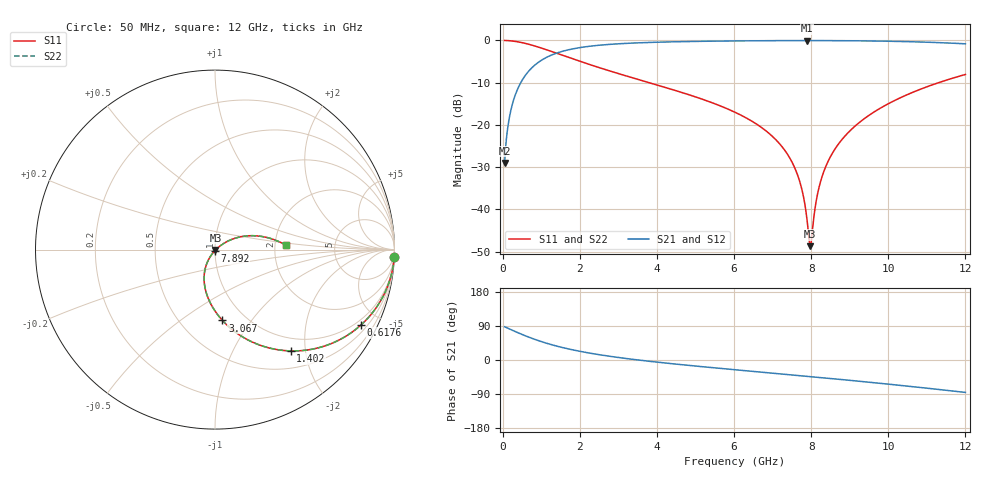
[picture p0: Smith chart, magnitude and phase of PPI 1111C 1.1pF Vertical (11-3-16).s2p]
# GHz S MA R 50
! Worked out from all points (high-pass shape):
!   1601 points, 50 MHz to 12 GHz, reference 50 ohm
!   highest |S21| = -0.04 dB at 7.892 GHz (marker M1); lowest = -29.0 dB at 50 MHz (marker M2)
!   |S21| within 3 dB of the highest: 1.389 GHz to end of sweep
!   lowest |S11| = -48.7 dB at 7.974 GHz (marker M3), VSWR 1.01, Z = 50.2 - j0.276 ohm
!   |S11| at or under -10 dB: 3.796 GHz to 11.31 GHz (7.509 GHz wide, 99.5 % of centre)
!   |S22| runs from -48.7 to 0.0 dB; largest |S21 - S12| = 0
!   S11 on the Smith chart (normalised r, x): 50 MHz: 1, -49; 617.6 MHz: 0.77, -3.98; 1.402 GHz: 0.77, -1.73; 3.067 GHz: 0.78, -0.73; 7.892 GHz: 1.00, -0.01; 12 GHz: 2.30, +0.13
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0.05  0.9994 -2.3  0.03551 87.7  0.03551 87.7  0.9994 -2.3
0.1545625  0.994 -7.2  0.1092 82.8  0.1092 82.8  0.994 -7.2
0.259125  0.9834 -11.9  0.1811 78.0  0.1811 78.0  0.9834 -11.9
0.617625  0.9152 -27.3  0.4024 62.7  0.4024 62.7  0.9152 -27.3
1.401844  0.7046 -53.2  0.7085 36.7  0.7085 36.7  0.7046 -53.2
2.044156  0.5581 -67.8  0.8283 22.1  0.8283 22.1  0.5581 -67.8
3.067375  0.3966 -84.0  0.9161 5.7  0.9161 5.7  0.3966 -84.0
4.038312  0.2934 -95.6  0.9536 -6.0  0.9536 -6.0  0.2934 -95.6
6.025  0.1411 -114.6  0.9869 -25.7  0.9869 -25.7  0.1411 -114.6
6.824156  0.08528 -121.0  0.9929 -33.1  0.9929 -33.1  0.08528 -121.0
7.361906  0.04665 -123.9  0.9952 -38.1  0.9952 -38.1  0.04665 -123.9
7.698  0.02179 -121.9  0.9958 -41.2  0.9958 -41.2  0.02179 -121.9
7.810031  0.01346 -116.8  0.9959 -42.2  0.9959 -42.2  0.01346 -116.8
7.892188  0.007586 -104.6  0.9959 -43.0  0.9959 -43.0  0.007586 -104.6
7.974344  0.003665 -48.6  0.9959 -43.8  0.9959 -43.8  0.003665 -48.6
8.019156  0.004865 -3.2  0.9959 -44.2  0.9959 -44.2  0.004865 -3.2
8.123719  0.012 26.7  0.9958 -45.2  0.9958 -45.2  0.012 26.7
8.220812  0.0195 32.7  0.9956 -46.1  0.9956 -46.1  0.0195 32.7
8.556906  0.04671 35.8  0.9945 -49.3  0.9945 -49.3  0.04671 35.8
9.139469  0.09688 32.5  0.9905 -55.0  0.9905 -55.0  0.09688 32.5
10.01331  0.1793 24.6  0.9785 -63.8  0.9785 -63.8  0.1793 24.6
12  0.3954 3.6  0.9118 -85.5  0.9118 -85.5  0.3954 3.6
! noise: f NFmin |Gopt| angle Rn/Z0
0.05  0.0009224  0.9658  1.916  0.006102
1.372  0.00432  0.7182  11.28  0.003004
2.701  0.006846  0.6596  18.12  0.003751
4.031  0.009134  0.6309  24.96  0.00444
5.36  0.01136  0.6173  31.6  0.005139
6.682  0.0136  0.6141  37.92  0.005896
8.012  0.01596  0.6188  43.95  0.006772
9.341  0.01851  0.63  49.66  0.00782
10.67  0.02134  0.6465  55.05  0.009113
12  0.02454  0.6676  60.17  0.01075
